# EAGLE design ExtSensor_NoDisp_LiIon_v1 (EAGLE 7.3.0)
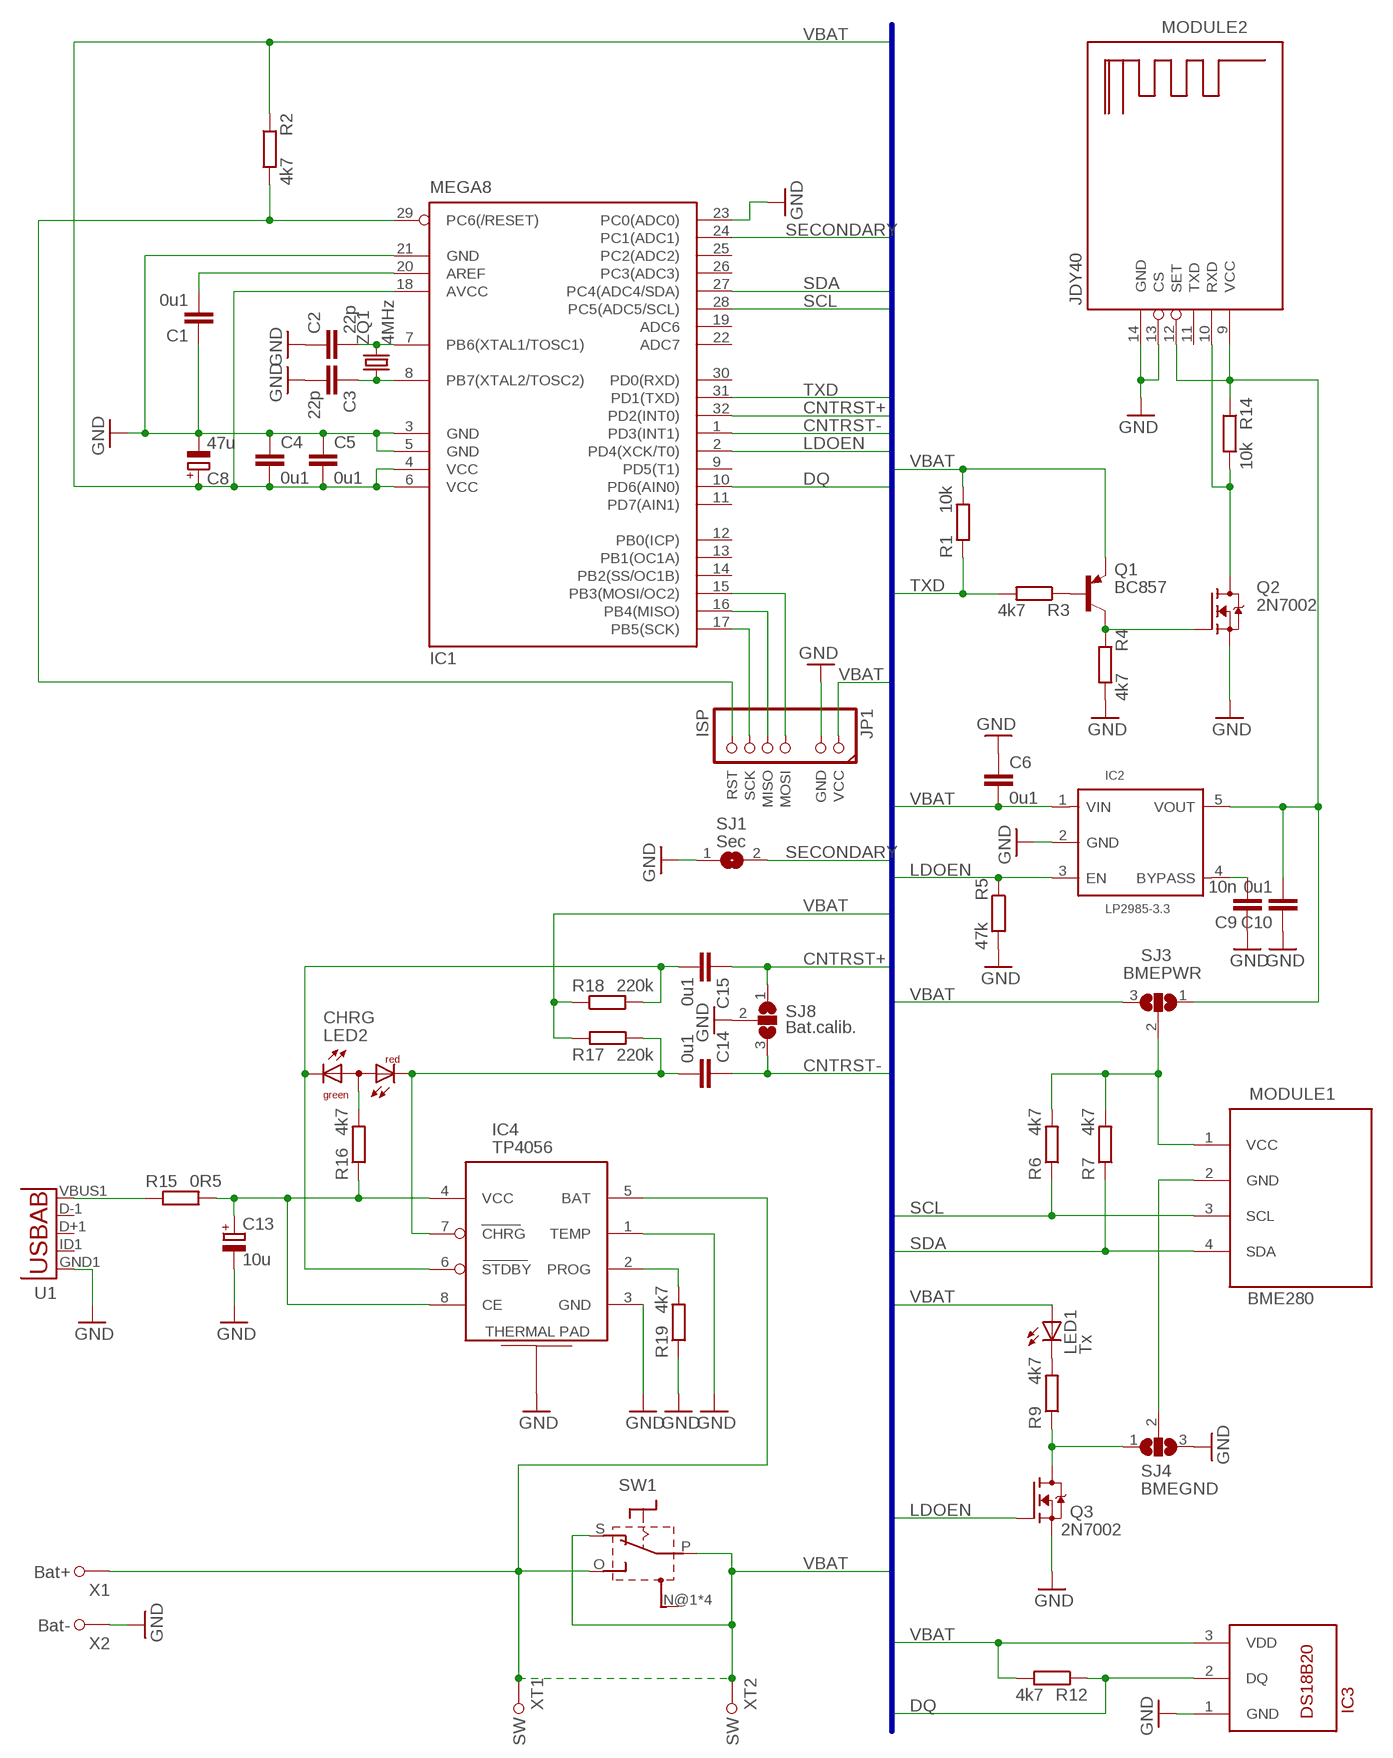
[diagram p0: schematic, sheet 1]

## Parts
C1  0u1  C-EUC0805T  [C0805T]
C2  22p  C-EUC0805T  [C0805T]
C3  22p  C-EUC0805T  [C0805T]
C4  0u1  C-EUC0805T  [C0805T]
C5  0u1  C-EUC0805T  [C0805T]
C6  0u1  C-EUC0805T  [C0805T]
C8  47u  CPOL-EUSMCB  [SMC_B]
C9  10n  C-EUC0805T  [C0805T]
C10  0u1  C-EUC0805T  [C0805T]
C13  10u  CPOL-EUSMCB  [SMC_B]
C14  0u1  C-EUC0805T  [C0805T]
C15  0u1  C-EUC0805T  [C0805T]
IC1  MEGA8  MEGA8-AI  [TQFP32-08]
IC2  LP2985-3.3  LP2985-XX  [SOT23-5]
IC3  DS18B20  DS18B20/-BH  [TO92-/BIG_HOLES]
IC4  TP4056  [SO08_POWER]
JP1  ISP  CONN1X7(2+4)_ISP+/P/NI  [1X07_ISP+POINTS_NO_INF]
LED1  Tx  LED3MM  [LED3MM]
LED2  CHRG  LED_DUO_RG_CA3MM  [LED_DUO-3MM]
MODULE1  BME280  BM(P|E)280_I2C/6  [BM(P|E)280_I2C_3V]
MODULE2  JDY40  JDY40_NO_GPIO/SMD  [JDY40_NG_SMD]
Q1  BC857  BC857THIN  [SOT23_THIN]
Q2  2N7002  2N7002/THIN  [SOT23_THIN]
Q3  2N7002  2N7002/THIN  [SOT23_THIN]
R1  10k  R-EU_R0805T  [R0805T]
R2  4k7  R-EU_R0805T  [R0805T]
R3  4k7  R-EU_R0805T  [R0805T]
R4  4k7  R-EU_R0805T  [R0805T]
R5  47k  R-EU_R0805T  [R0805T]
R6  4k7  R-EU_R0805T  [R0805T]
R7  4k7  R-EU_R0805T  [R0805T]
R9  4k7  R-EU_R0805T  [R0805T]
R12  4k7  R-EU_R0805T  [R0805T]
R14  10k  R-EU_R0805T  [R0805T]
R15  0R5  R-EU_R1206T  [R1206T]
R16  4k7  R-EU_R0805T  [R0805T]
R17  220k  R-EU_R0805T  [R0805T]
R18  220k  R-EU_R0805T  [R0805T]
R19  4k7  R-EU_R0805T  [R0805T]
SJ1  Sec  SJ  [SJ]
SJ3  BMEPWR  SJ2W  [SJ_2]
SJ4  BMEGND  SJ2W  [SJ_2]
SJ8  Bat.calib.  SJ2W  [SJ_2]
SW1  SLIDE_SWITCH  [SLIDE_SWITCH_2.7X6.6]
U1  USB5""  [USB-MICRO-SMD]
X1  Bat+  SIMPLE_WIRED_HOLE/1.0MM  [SIMPLE_WIRED_HOLE_1.0]
X2  Bat-  SIMPLE_WIRED_HOLE/1.0MM  [SIMPLE_WIRED_HOLE_1.0]
XT1  SW  SIMPLE_WIRED_HOLE/1.0MM  [SIMPLE_WIRED_HOLE_1.0]
XT2  SW  SIMPLE_WIRED_HOLE/1.0MM  [SIMPLE_WIRED_HOLE_1.0]
ZQ1  4MHz  CRYSTAL_AL/TH  [HC49/S]

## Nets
BMEGND: MODULE1.2(GND) SJ4.2
BMEPWR: MODULE1.1(VCC) R6.2 R7.2 SJ3.2
CNTRST+: C15.1 IC1.32(PD2(INT0)) SJ8.1
CNTRST-: C14.1 IC1.1(PD3(INT1)) SJ8.3
DQ: IC1.10(PD6(AIN0)) IC3.2(DQ) R12.1
GND: C1.1 C2.1 C3.2 C4.1 C5.1 C6.1 C8.- C9.1 C10.1 C13.- IC1.3(GND) IC1.5(GND) IC1.21(GND) IC1.23(PC0(ADC0)) IC2.2(GND) IC3.1(GND) IC4.1(TEMP) IC4.3(GND) IC4.THERMAL_PAD(THERMAL) JP1.GND MODULE2.13(CS) MODULE2.14(GND) Q2.2(S) Q3.2(S) R4.2 R5.2 R19.1 SJ1.1 SJ4.3 SJ8.2 U1.GND1(GND) X2.P$1
LDO_OUT: C10.2 IC2.5(VOUT) MODULE2.9(VCC) MODULE2.12(SET) R14.1 SJ3.1
LDOEN: IC1.2(PD4(XCK/T0)) IC2.3(EN) Q3.1(G) R5.1
MISO: IC1.16(PB4(MISO)) JP1.MISO
MOSI: IC1.15(PB3(MOSI/OC2)) JP1.MOSI
N$1: C3.1 IC1.8(PB7(XTAL2/TOSC2)) ZQ1.1
N$2: Q1.3(C) Q2.1(G) R4.1
N$3: C2.2 IC1.7(PB6(XTAL1/TOSC1)) ZQ1.2
N$4: C9.2 IC2.4(BYPASS)
N$5: C14.2 IC4.7(CHRG) LED2.COLOR1(CR) R17.2
N$6: R15.1 U1.VBUS1(VBUS)
N$7: LED1.K(C) R9.2
N$8: C13.+ IC4.4(VCC) IC4.8(CE) R15.2 R16.1
N$9: C15.2 IC4.6(STDBY) LED2.COLOR2(CG) R18.2
N$10: C1.2 IC1.20(AREF)
N$12: Q1.1(B) R3.1
N$13: IC4.2(PROG) R19.2
N$16: Q3.3(D) R9.1 SJ4.1
N$17: LED2.COMMON(A) R16.2
RST: IC1.29(PC6(/RESET)) JP1.RST R2.2
SCK: IC1.17(PB5(SCK)) JP1.SCK
SCL: IC1.28(PC5(ADC5/SCL)) MODULE1.3(SCL) R6.1
SDA: IC1.27(PC4(ADC4/SDA)) MODULE1.4(SDA) R7.1
SECONDARY: IC1.24(PC1(ADC1)) SJ1.2
TX_OUT: MODULE2.10(RXD) Q2.3(D) R14.2
TXD: IC1.31(PD1(TXD)) R1.1 R3.2
VBAT: C4.2 C5.2 C6.2 C8.+ IC1.4(VCC) IC1.6(VCC) IC1.18(AVCC) IC2.1(VIN) IC3.3(VDD) IC4.5(BAT) JP1.+5V(VCC) LED1.A Q1.2(E) R1.2 R2.1 R12.2 R17.1 R18.1 SJ3.3 SW1.O SW1.P SW1.S X1.P$1 XT1.P$1 XT2.P$1
Unconnected: IC1.9(PD5(T1)) IC1.11(PD7(AIN1)) IC1.12(PB0(ICP)) IC1.13(PB1(OC1A)) IC1.14(PB2(SS/OC1B)) IC1.19(ADC6) IC1.22(ADC7) IC1.25(PC2(ADC2)) IC1.26(PC3(ADC3)) IC1.30(PD0(RXD)) MODULE2.11(TXD) SW1.N@1(N) SW1.N@2(N) SW1.N@3(N) SW1.N@4(N) U1.D+1(D+) U1.D-1(D-) U1.ID1(USBID)

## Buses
VBAT,TXD,SCL,SDA,DQ,MOSI,SCK,LDOEN,CNTRST-,CNTRST+,TXEN,SECONDARY

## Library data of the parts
C1-C6 C9 C10 C14 C15 = rcl:C-EU: CAPACITOR, European symbol
C8 C13 = rcl:CPOL-EU: POLARIZED CAPACITOR, European symbol
IC1 = atmel:MEGA8: MICROCONTROLLER 8 Kbytes FLASH, 1 kbytes SRAM, 512 bytes EEPROM, USART, 6-channel 10 bit ADC, 2-channel 8 bit ADC Pin compatible with Atmega48, ATMega88, ATMega168 Source: avr.lbr; MPN: ATMEGA8-16AU; OC_FARNELL: 9171371; OC_NEWARK: 73M8863
IC2 = v-reg-AL:LP2985-XX: Texas Instruments LP2985 150-mA Low-noise Low-dropout Regulator With Shutdown
IC3 = misc-active-AL:DS18B20
IC4 = v-reg-AL:TP4056: TP4056 Standalone 1A Linear Li-lon Battery Charger with Thermal Regulation
JP1 = pinhead-AL:CONN1X7(2+4)_ISP+: PIN HEADER
LED1 = led-AL:LED
LED2 = led-AL:LED_DUO_RG_CA
MODULE1 = modules-external-AL:BM(P|E)280_I2C
MODULE2 = modules-external-AL:JDY40_NO_GPIO
Q1 = transistor-pnp-AL:BC857*: PNP Transistror
Q2 Q3 = transistor-fet-drv-AL:2N7002: Small signal N-Channel MOSFET transistor
R1-R7 R9 R12 R14-R19 = rcl:R-EU_: RESISTOR, European symbol
SJ1 = jumper:SJ: SMD solder JUMPER
SJ3 SJ4 SJ8 = jumper:SJ2W: SMD solder JUMPER
SW1 = switch-misc-AL:SLIDE_SWITCH
U1 = usb:USB5: This is a USB AB connector that is compatible with USB OTG. i.e. this connector can serve as a host or device
X1 X2 XT1 XT2 = connectors-AL:SIMPLE_WIRED_HOLE
ZQ1 = crystal:CRYSTAL_AL

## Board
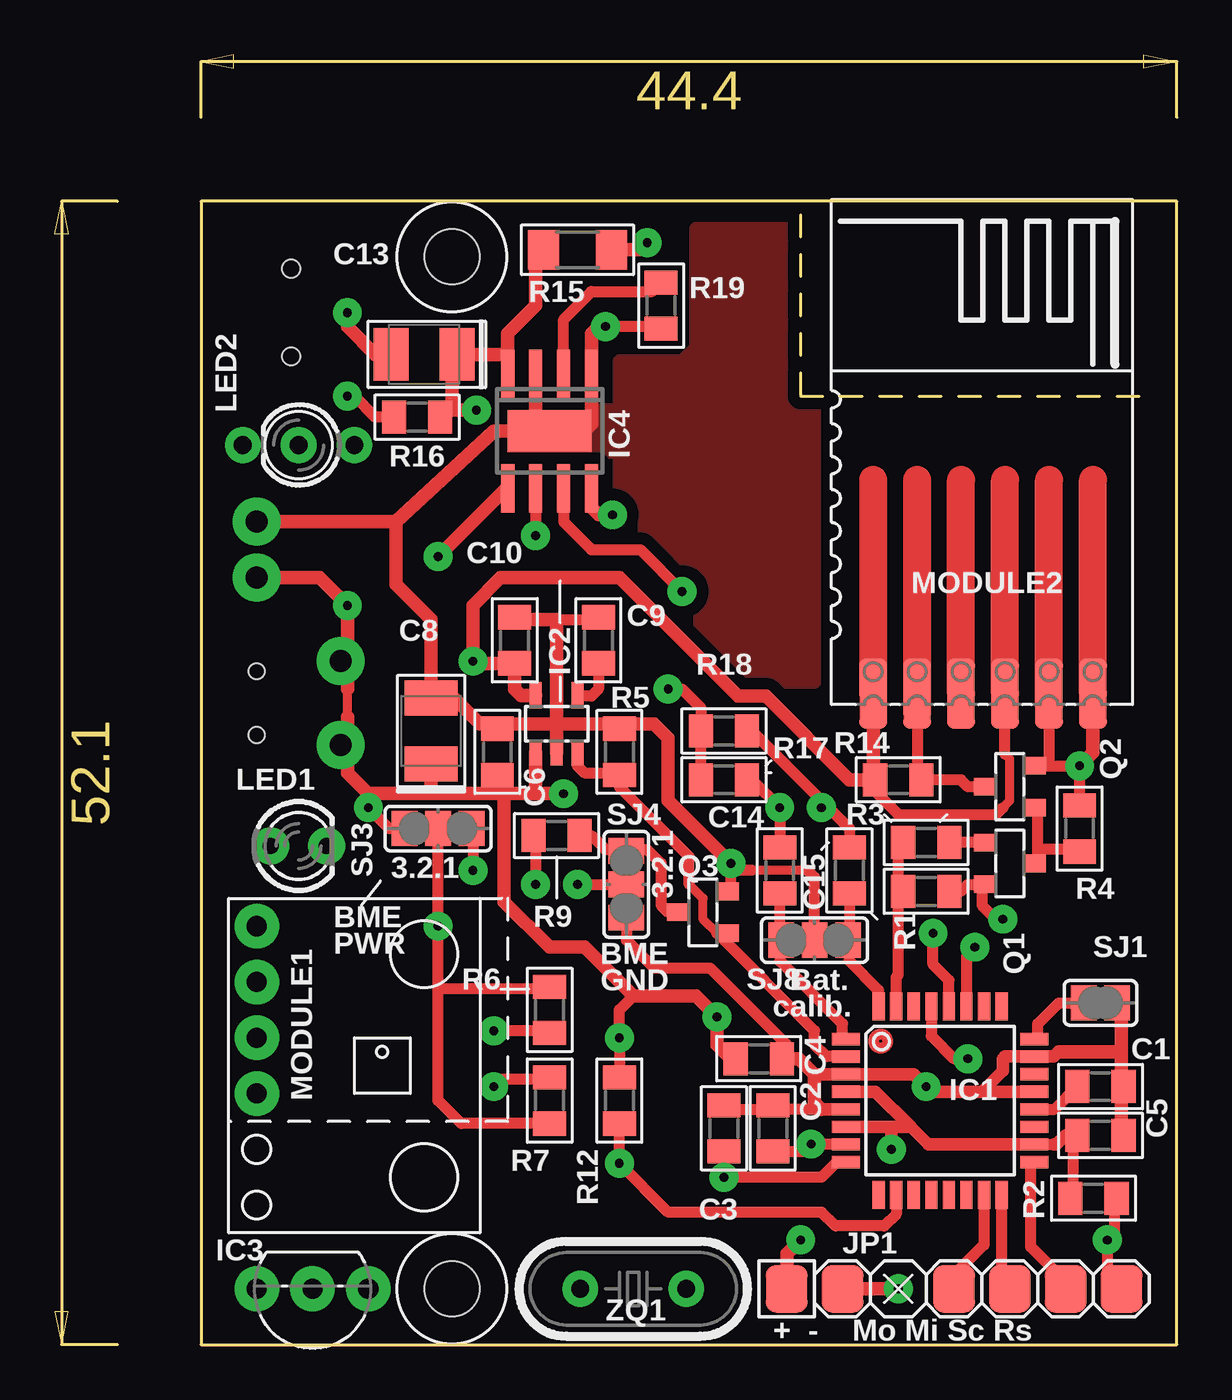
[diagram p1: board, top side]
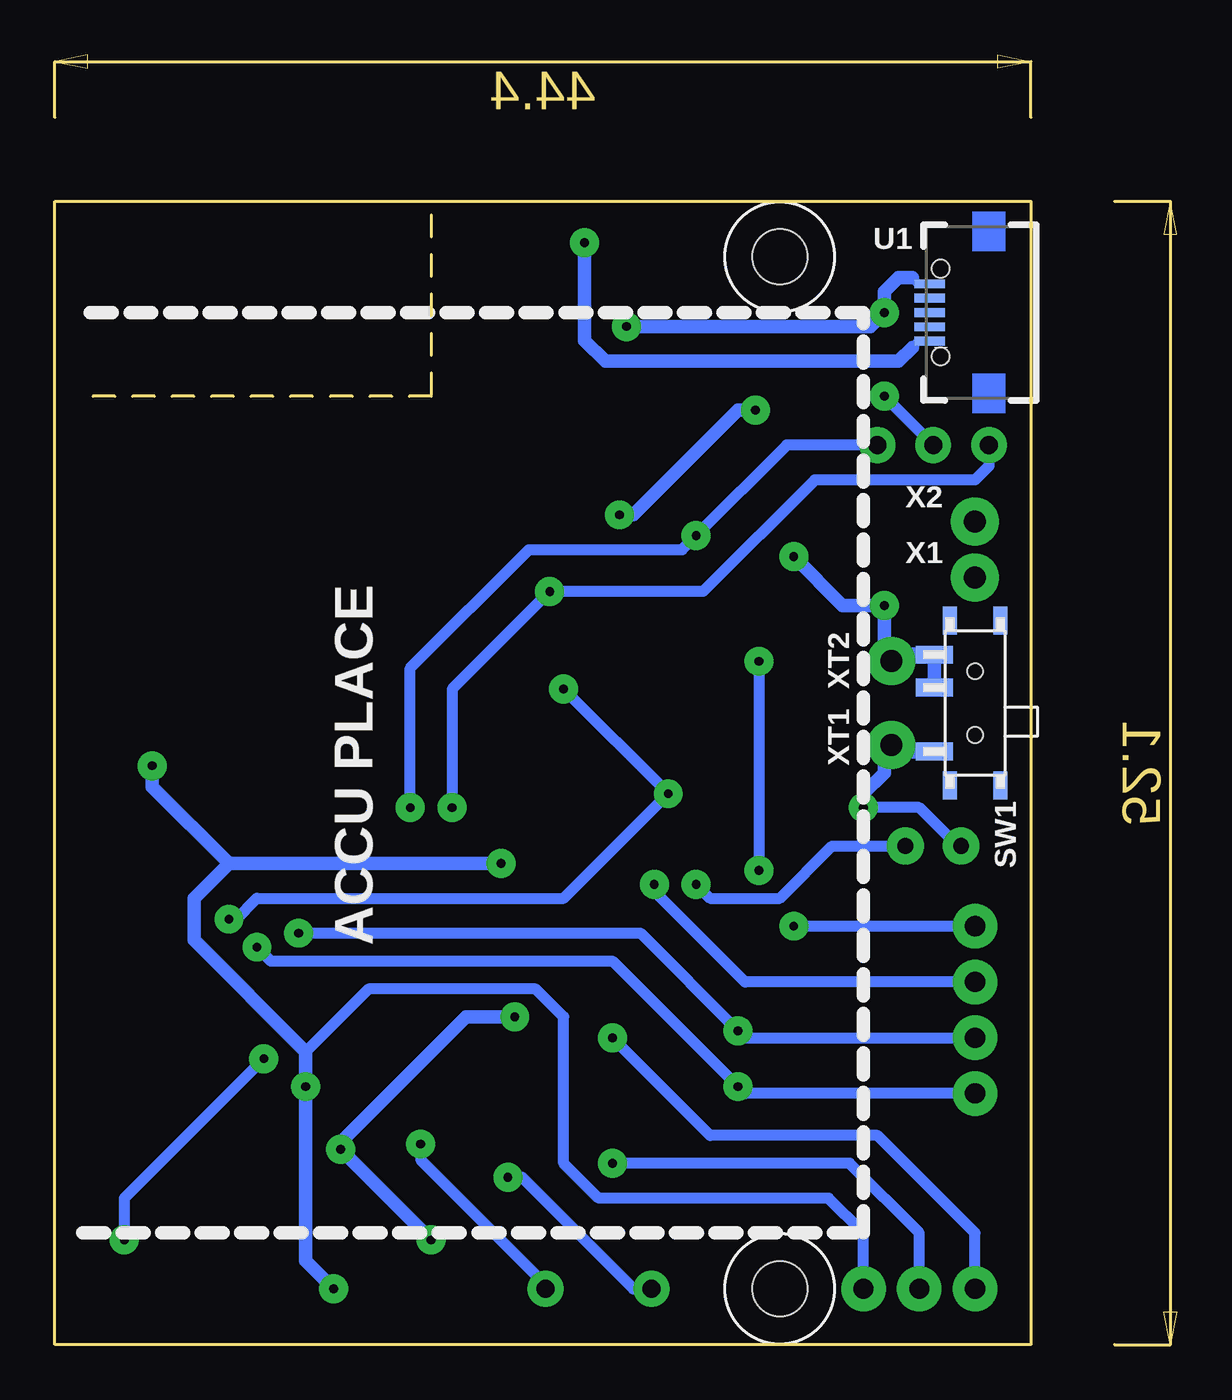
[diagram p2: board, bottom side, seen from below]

Size 51.09 x 58.72 mm. Coordinates in mm from the lower left corner, seen from the top.
Outline: 33.95,51.44 33.95,43.18 49.83,43.18
Outline: 6.65,0 51.09,0 51.09,52.06 6.65,52.06 6.65,0
Copper layers (1*16): Top 0.035mm / dielectric 1.5mm / Bottom 0.035mm
Design rules "default": minimum track width 12mil, minimum drill 14mil, track to track 8mil, track to pad 8mil, pad to pad 8mil, via to via 8mil, smd to smd 8mil, copper to edge 20mil, drill to drill 30mil, minimum pad ring 16mil, minimum via ring 18mil, stop-mask expansion 4mil, vias tented up to drill 0mil, thermal gap 16mil
Holes 2.5 mm at 18.08,49.53 18.08,2.54

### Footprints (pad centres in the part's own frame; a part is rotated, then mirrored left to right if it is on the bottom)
C0805T = smd 1.1 x 1.5: 1 -1.05,0; 2 1.05,0
SMC_B = smd 1.6 x 2.4: + -1.5,0; - 1.5,0
TQFP32-08 = smd 1.27 x 0.559: 1 -4.293,2.8; 2 -4.293,2; 3 -4.293,1.2; 4 -4.293,0.4; 5 -4.293,-0.4; 6 -4.293,-1.2; 7 -4.293,-2; 8 -4.293,-2.8; 17 4.293,-2.8; 18 4.293,-2; 19 4.293,-1.2; 20 4.293,-0.4; 21 4.293,0.4; 22 4.293,1.2; 23 4.293,2; 24 4.293,2.8 | smd 0.559 x 1.27: 9 -2.8,-4.293; 10 -2,-4.293; 11 -1.2,-4.293; 12 -0.4,-4.293; 13 0.4,-4.293; 14 1.2,-4.293; 15 2,-4.293; 16 2.8,-4.293; 25 2.8,4.293; 26 2,4.293; 27 1.2,4.293; 28 0.4,4.293; 29 -0.4,4.293; 30 -1.2,4.293; 31 -2,4.293; 32 -2.8,4.293
SOT23-5 = smd 0.55 x 1.2: 1 -0.95,-1.3; 2 0,-1.3; 3 0.95,-1.3; 4 0.95,1.3; 5 -0.95,1.3
TO92-/BIG_HOLES = drill 0.914 pad 2.032: 1 -2.54,0; 2 0,0; 3 2.54,0
SO08_POWER = smd 0.6 x 2.2: 1 -1.905,-2.6; 2 -0.635,-2.6; 3 0.635,-2.6; 4 1.905,-2.6; 5 1.905,2.6; 6 0.635,2.6; 7 -0.635,2.6; 8 -1.905,2.6 | smd 3.81 x 1.93: THERMAL_PAD 0,0
1X07_ISP+POINTS_NO_INF = smd 1.905 x 2.159: +5V -7.62,0; GND -5.08,0; MISO 2.54,0; MOSI 0,0; RST 7.62,0; SCK 5.08,0
LED3MM = drill 0.711 pad 1.676: A -1.27,0; K 1.27,0
LED_DUO-3MM = drill 0.813: COLOR1 2.54,0; COLOR2 -2.54,0; COMMON 0,0
BM(P|E)280_I2C_3V = drill 0.914 pad 2.032: 1 6.35,3.81; 2 3.81,3.81; 3 1.27,3.81; 4 -1.27,3.81
JDY40_NG_SMD = smd 1.27 x 3.175: 9 -4.95,-11; 10 -2.95,-11; 11 -0.95,-11; 12 1.05,-11; 13 3.05,-11; 14 5.05,-11
SOT23_THIN = smd 0.8 x 1.1: 1 -0.95,-1.1; 2 0.95,-1.1; 3 0,1.1
R0805T = smd 1.1 x 1.5: 1 -1.05,0; 2 1.05,0
R1206T = smd 1.4 x 1.8: 1 -1.55,0; 2 1.55,0
SJ = smd 1.168 x 1.6: 1 -0.762,0; 2 0.762,0
SJ_2 = smd 1.168 x 1.6: 1 -1.524,0; 2 0,0; 3 1.524,0
SLIDE_SWITCH_2.7X6.6 = smd 1.27 x 0.635: N@1 -3.75,-1.15; N@2 -3.75,1.15; N@3 3.75,1.15; N@4 3.75,-1.15 | smd 0.813 x 1.676: O 2.2,-1.85; P -0.7,-1.85; S -2.2,-1.85 | hole 0.71: -1.45,0; 1.45,0
USB-MICRO-SMD = smd 1.4 x 0.4: D+1 2.7,0; D-1 2.7,0.65; GND1 2.7,-1.3; ID1 2.7,-0.65; VBUS1 2.7,1.3 | hole 0.8: 2.2,2; 2.2,-2
SIMPLE_WIRED_HOLE_1.0 = drill 1 pad 2.184: P$1 0,0
HC49/S = drill 0.813: 1 -2.413,0; 2 2.413,0

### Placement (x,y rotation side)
C1  47.61,11.75 180 top
C2  32.69,9.84 270 top
C3  30.46,9.84 90 top
C4  32.05,13.02 180 top
C5  47.61,9.52 180 top
C6  20.14,26.99 270 top
C8  17.13,27.94 90 top
C9  24.75,32.07 270 top
C10  20.94,32.07 270 top
C13  16.81,45.09 180 top
C14  33,21.59 90 top
C15  36.18,21.59 90 top
IC1  40.31,11.11 0 top
IC2  22.84,28.26 0 top
IC3  11.73,2.54 180 top
IC4  22.53,41.59 180 top
JP1  40.94,2.54 0 top
LED1  11.1,22.7 0 top
LED2  11.1,40.96 180 top
MODULE1  13,12.7 90 top
MODULE2  42.21,40.64 0 top
Q1  43.48,21.91 270 top
Q2  43.48,25.4 90 top
Q3  29.51,19.68 90 top
R1  39.67,20.64 0 top
R2  47.29,6.67 0 top
R3  39.67,22.86 180 top
R4  46.66,23.49 90 top
R5  25.7,26.99 90 top
R6  22.53,15.24 90 top
R7  22.53,11.11 270 top
R9  22.84,23.18 180 top
R12  25.7,11.11 90 top
R14  38.4,25.72 0 top
R15  23.79,49.85 180 top
R16  16.49,42.23 180 top
R17  30.46,25.72 0 top
R18  30.46,27.94 0 top
R19  27.61,47.31 90 top
SJ1  47.61,15.56 180 top
SJ3  17.45,23.49 180 top
SJ4  26.02,20.95 270 top
SJ8  34.59,18.41 180 top
SW1  9.19,29.21 270 bottom
U1  8.55,46.99 180 bottom
X1  9.19,34.92 0 bottom
X2  9.19,37.46 0 bottom
XT1  13,27.3 0 bottom
XT2  13,31.12 0 bottom
ZQ1  26.34,2.54 0 top

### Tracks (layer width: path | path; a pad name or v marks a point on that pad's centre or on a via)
BMEGND  (via drill 0.4)
  Top 0.508: v23.79,20.95 SJ4.2
  Bottom 0.508: MODULE1.2 19.67,16.51 23.79,20.64 v23.79,20.95
BMEPWR  (via drill 0.4)
  Top 0.508: SJ3.2 v17.45,19.05 17.45,16.19 | R7.2 18.5,10.06 17.45,11.11 17.45,16.19 | R6.2 22.21,16.19 17.45,16.19
  Bottom 0.508: MODULE1.1 v17.45,19.05
CNTRST+
  Top 0.508: C15.1 36.18,18.41 | SJ8.1 36.18,18.41 | IC1.32 37.5,16.13 36.18,17.46 36.18,18.41
CNTRST-
  Top 0.508: IC1.1 35.92,13.91 35.86,13.97 35.86,14.61 33,17.46 33,18.41 | 33,18.41 C14.1 | SJ8.3 33,18.41
DQ  (via drill 0.4)
  Top 0.508: IC1.10 38.31,5.94 37.77,5.4 35.54,5.4 34.91,6.03 27.92,6.03 v25.7,8.25 R12.1
  Bottom 0.508: IC3.2 11.73,5.08 14.91,8.25 v25.7,8.25
GND  (via drill 0.4)
  Top 0.406: 34.27,21.59 31.73,21.59
  Top 0.508: C3.2 30.46,10.72 32.69,10.72 | C2.1 32.69,10.72 | 34.91,10.71 32.76,10.71 32.69,10.72 | 22.84,33.02 24.65,33.02 C9.1 | 25.07,28.26 25.48,28.26 R5.2 | SJ8.2 34.59,21.27 34.27,21.59 | 31.73,21.59 30.78,21.59 | Q3.2 30.78,20.63 30.78,20.64 30.78,21.59 | 30.78,21.59 v30.78,21.91 | SJ4.3 26.02,18.41 27.29,17.14 29.83,17.14 33.32,13.65 33.32,13.11 C4.1 | Q2.2 44.75,26.35 45.07,26.35 45.26,26.35 | 45.26,26.35 v46.66,26.35 R4.2 | MODULE2.13 45.26,29.08 45.26,26.35 | R19.1 27.61,46.35 v25.07,46.35
  Top 0.559: IC1.5 34.91,10.71 | 34.59,12.31 IC1.3 39.11,12.31 v39.67,11.75 39.91,11.51 42.21,11.51 | IC1.21 42.21,11.51 | 42.21,11.51 43.16,12.46 43.16,13.02 43.26,13.11 IC1.23 45.48,13.11 45.7,13.34
  Top 0.61: 34.91,10.71 34.91,10.72 34.59,11.03 34.59,12.31 33.89,13.02 C4.1 | v38.4,2.54 JP1.GND | X2.P$1 15.54,37.46 | 15.54,37.46 15.54,34.61 17.13,33.02 C8.- 17.13,29.53 18.08,29.53 19.35,28.26 20.14,28.26 | IC2.2 22.84,28.26 | 22.84,28.26 22.84,33.02 20.94,33.02 C10.1 | 20.14,28.26 22.84,28.26 | C6.1 20.14,28.26 | 22.84,28.26 25.07,28.26 | v30.78,21.91 27.92,24.77 27.92,27.62 27.29,28.26 25.48,28.26 | MODULE2.14 47.26,26.96 v46.66,26.35 | v13.32,46.99 13.32,46.35 14.59,45.09 C13.- 15.54,45.72 | IC4.3 21.89,41.59 | 15.54,37.46 19.98,41.59 21.89,41.59 | 45.7,13.34 48.56,13.34 | 48.56,13.34 48.56,11.75 | 48.56,11.75 48.56,9.62 C5.1 | C1.1 48.56,11.75 | 48.56,13.34 48.56,15.37 SJ1.1 | v25.07,46.35 24.75,46.35 24.43,46.04 IC4.1 24.43,41.91 24.11,41.59 IC4.THERMAL_PAD 21.89,41.59
  Top 1.27: 45.26,29.08 45.26,39.37 | MODULE2.14 47.26,39.37
  Bottom 0.406: U1.GND1 11.76,48.29 12.05,48.58
  Bottom 0.508: IC3.1 14.27,5.08 15.86,6.67 26.34,6.67 27.92,8.25 27.92,14.92 29.19,16.19 36.81,16.19 39.67,13.34
  Bottom 0.61: 43.16,21.91 44.75,20.32 44.75,18.41 39.67,13.34 v39.67,11.75 39.67,3.81 v38.4,2.54 | 43.16,21.91 v30.78,21.91 | v46.66,26.35 46.66,25.4 43.16,21.91 | 12.05,48.58 12.68,48.58 13.32,47.94 v13.32,46.99 13.95,46.35 v25.07,46.35
  pour Top (isolate 0.533, no thermals): 24.43,40.64 25.7,40.64 25.7,35.24 30.78,30.16 34.59,30.16 34.59,50.8 29.19,50.8 29.19,45.4 28.56,44.77 25.7,44.77 25.7,42.55 24.43,42.55
LDO_OUT  (via drill 0.4)
  Top 0.406: 43.16,24.45 43.48,24.77 43.48,26.67 43.26,26.89
  Top 0.508: 19.13,31.02 v19.03,31.12 | SJ3.1 19.03,23.49 v19.03,21.59 | R14.1 37.26,26.12 37.26,25.27 38.4,24.13 42.84,24.13 43.16,24.45 | 43.26,26.89 MODULE2.12
  Top 0.61: IC2.5 21.22,29.56 20.94,29.84 C10.2 19.13,31.02 | v19.03,31.12 19.03,33.66 20.3,34.92 25.7,34.92 31.1,29.53 32.37,29.53 36.18,25.72 R14.1 | MODULE2.9 37.26,26.12
  Top 1.27: MODULE2.9 37.26,39.37 | MODULE2.12 43.26,39.37
  Bottom 0.508: v19.03,31.12 v19.03,21.59
LDOEN
  Top 0.406: 30.14,18.73 29.51,19.37 29.51,20.32 28.88,20.95
  Top 0.508: IC2.3 23.79,26.35 24.11,26.03 25.7,26.03 R5.1 25.7,25.4 28.88,22.22 28.88,20.95 | IC1.2 35.13,13.11 34.59,13.65 34.59,14.29 30.14,18.73 30.46,18.73 Q3.1
MISO
  Top 0.508: IC1.16 43.11,2.91 JP1.MISO
MOSI
  Top 0.508: IC1.15 42.31,4.54 40.94,3.17 JP1.MOSI
N$1  (via drill 0.4)
  Top 0.508: IC1.8 35.6,8.31 34.91,7.62 v30.46,7.62 C3.1
  Bottom 0.508: ZQ1.1 24.75,2.54 29.83,7.62 v30.46,7.62
N$2
  Top 0.508: Q1.3 44.75,21.91 44.75,22.54 | 44.75,22.54 44.75,24.45 Q2.1 | R4.1 46.66,22.54 44.75,22.54
N$3  (via drill 0.4)
  Top 0.508: IC1.7 34.42,9.11 | C2.2 34.1,8.79 34.42,9.11 | 34.42,9.11 v34.43,9.13
  Bottom 0.508: ZQ1.2 28.75,2.73 34.43,8.41 v34.43,9.13
N$4
  Top 0.508: C9.2 24.75,29.84 24.43,29.53 23.82,29.53 IC2.4
N$5  (via drill 0.4)
  Top 0.508: C14.2 v33,24.45 31.73,25.72 R17.2 | IC4.7 23.16,37.46 24.43,36.2 26.65,36.2 v28.56,34.29
  Bottom 0.508: v33,24.45 33,29.84 v28.56,34.29 21.57,34.29 16.49,39.37 9.19,39.37 8.55,40.01 LED2.COLOR1
N$6  (via drill 0.4)
  Top 0.61: R15.1 26.65,49.85 v26.97,50.16
  Bottom 0.406: 12.05,45.4 11.76,45.69 U1.VBUS1
  Bottom 0.61: v26.97,50.16 26.97,45.72 26.02,44.77 12.68,44.77 12.05,45.4
N$7  (via drill 0.4)
  Top 0.508: R9.2 21.89,22.86 v21.89,20.95
  Bottom 0.508: v21.89,20.95 21.25,20.32 18.08,20.32 15.7,22.7 LED1.K
N$8  (via drill 0.4)
  Top 0.508: R16.1 17.76,42.23 18.08,42.55
  Top 0.61: 20.62,45.09 C13.+ 18.08,45.72 18.08,42.55 v19.19,42.55 | 20.62,45.09 IC4.4 | IC4.8 24.43,38.1 24.75,37.78 v25.38,37.78 | R15.2 21.89,49.85 21.89,47.31 20.62,46.04 20.62,45.09
  Bottom 0.61: v25.38,37.78 24.75,37.78 19.98,42.55 v19.19,42.55
N$9  (via drill 0.4)
  Top 0.508: R18.2 31.73,27.94 34.91,24.77 v34.91,24.45 35.22,24.45 36.18,23.49 C15.2 | IC4.6 v21.89,36.83
  Bottom 0.508: v34.91,24.45 34.91,30.8 29.51,36.2 22.53,36.2 v21.89,36.83 17.76,40.96 LED2.COLOR2
N$10
  Top 0.508: IC1.20 45.52,10.71 C1.2
N$11
  Top 1.27: 41.26,29.64 41.26,39.37
N$12
  Top 0.508: Q1.1 42.21,22.86 R3.1
N$13
  Top 0.508: IC4.2 23.16,46.67 24.43,47.94 27.19,47.94 R19.2 27.61,48.26
N$16
  Top 0.508: R9.1 24.43,23.18 25.07,22.54 26.02,22.54 | 26.02,22.54 26.97,22.54 27.61,21.91 27.61,20 27.92,19.68 Q3.3 | SJ4.1 26.02,22.54
N$17  (via drill 0.4)
  Top 0.508: R16.2 14.59,42.23 13.64,43.18 v13.32,43.18
  Bottom 0.508: v13.32,43.18 LED2.COMMON
RST  (via drill 0.4)
  Top 0.508: JP1.RST 47.92,3.17 v47.92,4.76 48.24,5.08 48.24,6.67 R2.2 | IC1.29 39.91,14.05 40.94,13.02 v41.58,13.02
  Bottom 0.508: v41.58,13.02 47.92,6.67 v47.92,4.76
SCK
  Top 0.508: IC1.17 44.43,8.15 44.43,4.45 46.02,2.86 JP1.SCK
SCL  (via drill 0.4)
  Top 0.508: IC1.28 40.7,16.59 39.99,17.3 v39.99,18.73 | R6.1 22.21,14.29 v19.98,14.29
  Bottom 0.508: v39.99,18.73 24.43,18.73 v19.98,14.29 19.67,13.97 MODULE1.3
SDA  (via drill 0.4)
  Top 0.508: v41.89,18.1 41.5,17.69 IC1.27 | R7.1 22.21,12.06 20.3,12.06 v19.98,11.75
  Bottom 0.508: v41.89,18.1 41.26,17.46 25.7,17.46 v19.98,11.75 19.67,11.43 MODULE1.4
SECONDARY
  Top 0.508: IC1.24 44.69,13.91 44.75,13.97 44.75,14.61 45.7,15.56 SJ1.2
TX_OUT
  Top 0.508: Q2.3 41.58,25.4 41.26,25.72 R14.2 39.26,25.91 39.26,28.78 MODULE2.10
  Top 1.27: 39.26,28.78 39.26,39.37
TXD
  Top 0.508: IC1.31 38.31,16.73 38.4,16.83 38.4,20.64 | 38.4,20.64 38.4,22.96 R3.2 | R1.1 38.4,20.64
VBAT  (via drill 0.4)
  Top 0.406: 13.32,28.58 13.32,29.84
  Top 0.508: IC1.18 45.48,9.11 | R2.1 46.34,6.89 46.34,9.3 C5.2 | v27.92,29.84 28.56,29.84 29.41,28.99 R18.1 R17.1 | SJ3.3 15.22,23.49 v14.27,24.45 | 42.21,20.96 42.21,20.95 | v43.16,19.37 42.84,19.37 42.21,20 42.21,20.96 | R1.2 41.26,20.64 41.58,20.95 Q1.2 42.21,20.96 | R12.2 v25.7,13.97 25.7,15.24 26.34,15.88
  Top 0.559: IC1.4 37.36,11.51 38.97,9.91 | IC1.18 39.77,9.11 38.97,9.91 | IC1.6 38.08,9.91 | 38.08,9.91 38.97,9.91 | v38.08,8.89 38.08,9.91 | 45.48,9.11 45.61,9.11 46.02,9.52 C5.2
  Top 0.61: C4.2 30.78,13.02 30.14,13.65 v30.14,14.92 29.19,15.88 26.34,15.88 24.11,18.1 22.53,18.1 20.46,20.16 20.46,25.08 | C8.+ 17.13,25.08 | 17.13,25.08 14.27,25.08 | 14.27,25.08 13.32,26.03 13.32,27.3 | 14.27,25.08 v14.27,24.45 | 20.14,25.08 17.13,25.08 | C6.2 20.14,25.08 | 20.14,25.08 20.46,25.08 | 20.46,25.08 21.89,25.08 | 21.89,25.08 v23.16,25.08 | IC2.1 21.89,25.4 21.89,25.08 | X1.P$1 12.05,34.92 v13.32,33.66 13.32,31.43 | 13.32,27.3 13.32,28.58 | 13.32,29.84 13.32,31.43 | 12.37,31.43 13,31.43 | 13,31.43 13.32,31.43 | IC4.5 20.56,38.99 v17.45,35.88 | v33.95,4.76 33.32,4.13 JP1.+5V | XT2.P$1 13,31.43 | XT1.P$1 13.32,27.3
  Bottom 0.508: LED1.A 9.98,22.7 11.73,24.45 v14.27,24.45 | v27.92,29.84 v23.16,25.08 27.92,20.32 41.89,20.32 42.84,19.37 v43.16,19.37 | IC3.3 9.19,5.08 13.64,9.52 21.25,9.52 v25.7,13.97
  Bottom 0.61: v30.14,14.92 32.37,14.92 38.08,9.21 v38.08,8.89 v33.95,4.76 | v17.45,35.88 15.22,33.66 v13.32,33.66 13.32,31.75 13,31.43 11.1,31.43 11.07,31.41 SW1.S SW1.P | SW1.O 11.07,27.01 11.1,26.99 12.05,26.99 12.37,27.3 13.32,27.3 13.32,26.03 14.27,25.08 v14.27,24.45
(copper drawn outside any net)
  shapes: Top circle x1

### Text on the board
tPlace: 3.2.1 | 3.2.1 | BME / PWR | BME / GND | Bat. / calib. | + - Mo Mi Sc Rs
bPlace: ACCU PLACE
